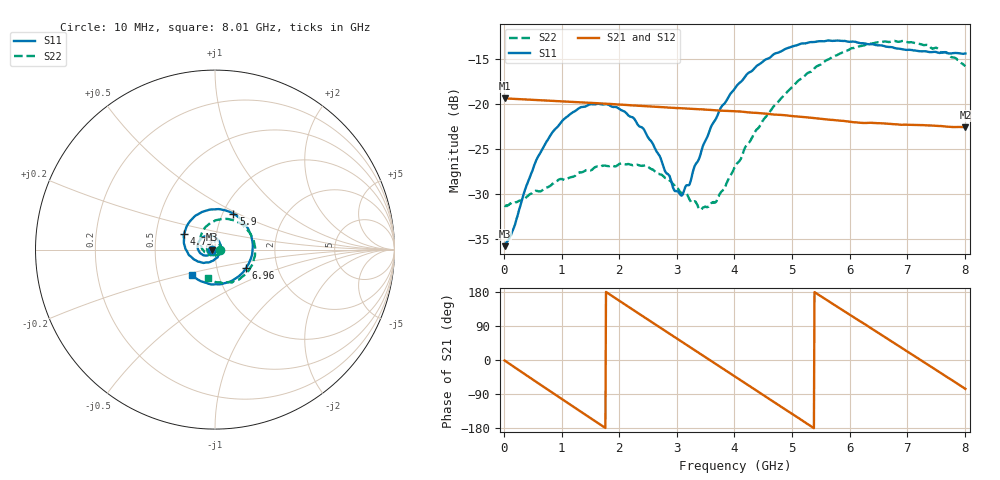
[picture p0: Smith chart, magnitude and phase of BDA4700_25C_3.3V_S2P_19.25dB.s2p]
!Agilent Technologies,E5071B,MY42404982,A.09.10
!Date: Mon Oct 20 18:11:08 2025
!Data & Calibration Information:
!Freq	S11:SOLT2(ON)	S21:SOLT2(ON)	S12:SOLT2(ON)	S22:SOLT2(ON)
# Hz S RI R 50
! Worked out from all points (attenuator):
!   801 points, 10 MHz to 8.01 GHz, reference 50 ohm
!   highest |S21| = -19.33 dB at 10 MHz (marker M1); lowest = -22.6 dB at 8.01 GHz (marker M2)
!   lowest |S11| = -35.8 dB at 10 MHz (marker M3), VSWR 1.03, Z = 48.4 - j0.109 ohm
!   |S11| at or under -10 dB: start of sweep to end of sweep
!   |S22| runs from -31.8 to -12.9 dB; largest |S21 - S12| = 0.0012
!   S11 on the Smith chart (normalised r, x): 10 MHz: 0.97, -0.00; 4.73 GHz: 0.70, +0.12; 5.9 GHz: 1.12, +0.47; 6.96 GHz: 1.39, -0.29; 8.01 GHz: 0.75, -0.22
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1e7  -0.0161 -0.00112  0.108 -0.00236  0.108 -0.00242  0.0272 -0.000845
1.5e8  -0.0172 -0.0096  0.1031 -0.0291  0.103 -0.0292  0.0272 -0.00743
4e8  -0.0259 -0.0246  0.0795 -0.0704  0.0795 -0.0704  0.0213 -0.0219
7e8  -0.0484 -0.0334  0.0323 -0.0999  0.0323 -0.0999  0.00564 -0.0333
1.02e9  -0.0778 -0.0237  -0.0262 -0.1004  -0.0261 -0.1004  -0.0169 -0.0341
1.35e9  -0.0963 0.00613  -0.0761 -0.0684  -0.0761 -0.0685  -0.0379 -0.0173
2.08e9  -0.0505 0.0763  -0.0845 0.0519  -0.0845 0.0518  -0.0285 0.0363
2.42e9  -0.00554 0.0727  -0.0405 0.0888  -0.0404 0.0888  -0.00186 0.0453
2.68e9  0.0217 0.048  0.0024 0.0965  0.00222 0.0965  0.0165 0.0374
2.95e9  0.0317 0.0102  0.0451 0.084  0.045 0.0838  0.0284 0.0211
3.09e9  0.029 -0.0108  0.0638 0.0702  0.0631 0.0705  0.0305 0.00934
3.4e9  0.00206 -0.051  0.0894 0.0277  0.0896 0.0278  0.0216 -0.0141
3.54e9  -0.0182 -0.0644  0.0929 0.00537  0.0929 0.00516  0.0128 -0.0235
3.69e9  -0.0448 -0.0714  0.0905 -0.0185  0.0905 -0.0188  -0.000742 -0.0288
4.01e9  -0.1069 -0.0601  0.0663 -0.0628  0.0663 -0.0626  -0.035 -0.0279
4.73e9  -0.1729 0.0856  -0.0373 -0.079  -0.0369 -0.0792  -0.0828 0.0574
5.35e9  -0.0627 0.213  -0.0837 -0.00465  -0.0837 -0.00509  -0.0143 0.1529
5.9e9  0.103 0.2005  -0.0508 0.0625  -0.051 0.0622  0.1137 0.1589
6.68e9  0.2079 -0.0156  0.046 0.0625  0.0462 0.0625  0.2223 -0.0072
6.96e9  0.174 -0.101  0.0685 0.0347  0.0686 0.0342  0.2082 -0.0836
7.48e9  0.0322 -0.1931  0.0692 -0.0311  0.0692 -0.0312  0.0977 -0.1811
8.01e9  -0.1279 -0.1429  0.0177 -0.0723  0.018 -0.0723  -0.0381 -0.1584
